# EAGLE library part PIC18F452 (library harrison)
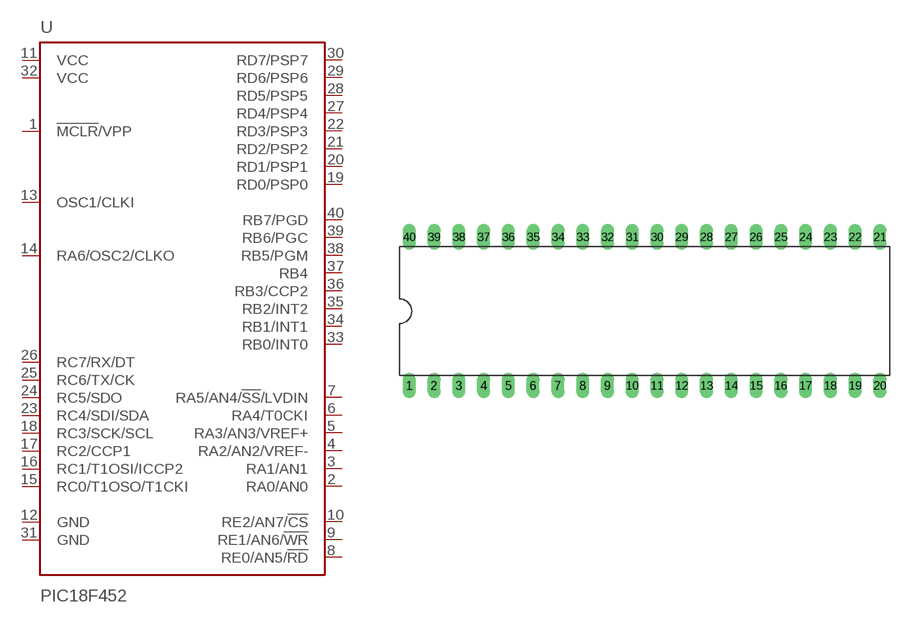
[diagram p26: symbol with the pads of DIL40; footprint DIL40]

Designator prefix U

## PIC18F452  [DIL40]
1  !MCLR!/VPP  in
2  RA0/AN0
3  RA1/AN1
4  RA2/AN2/VREF-
5  RA3/AN3/VREF+
6  RA4/T0CKI
7  RA5/AN4/!SS!/LVDIN
8  RE0/AN5/!RD
9  RE1/AN6/!WR
10  RE2/AN7/!CS
11  VCC  pwr
12  GND  pwr
13  OSC1/CLKI  in
14  RA6/OSC2/CLKO  out
15  RC0/T1OSO/T1CKI
16  RC1/T1OSI/ICCP2
17  RC2/CCP1
18  RC3/SCK/SCL
19  RD0/PSP0
20  RD1/PSP1
21  RD2/PSP2
22  RD3/PSP3
23  RC4/SDI/SDA
24  RC5/SDO
25  RC6/TX/CK
26  RC7/RX/DT
27  RD4/PSP4
28  RD5/PSP5
29  RD6/PSP6
30  RD7/PSP7
31  GND  pwr
32  VCC  pwr
33  RB0/INT0
34  RB1/INT1
35  RB2/INT2
36  RB3/CCP2
37  RB4
38  RB5/PGM
39  RB6/PGC
40  RB7/PGD

## Footprint DIL40 (pad centres in mm)
drill 0.813 long: 1 -22.86,-7.62; 2 -20.32,-7.62; 3 -17.78,-7.62; 4 -15.24,-7.62; 5 -12.7,-7.62; 6 -10.16,-7.62; 7 -7.62,-7.62; 8 -5.08,-7.62; 9 -2.54,-7.62; 10 0,-7.62; 11 2.54,-7.62; 12 5.08,-7.62; 13 7.62,-7.62; 14 10.16,-7.62; 15 12.7,-7.62; 16 15.24,-7.62; 17 17.78,-7.62; 18 20.32,-7.62; 19 22.86,-7.62; 20 25.4,-7.62; 21 25.4,7.62; 22 22.86,7.62; 23 20.32,7.62; 24 17.78,7.62; 25 15.24,7.62; 26 12.7,7.62; 27 10.16,7.62; 28 7.62,7.62; 29 5.08,7.62; 30 2.54,7.62; 31 0,7.62; 32 -2.54,7.62; 33 -5.08,7.62; 34 -7.62,7.62; 35 -10.16,7.62; 36 -12.7,7.62; 37 -15.24,7.62; 38 -17.78,7.62; 39 -20.32,7.62; 40 -22.86,7.62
